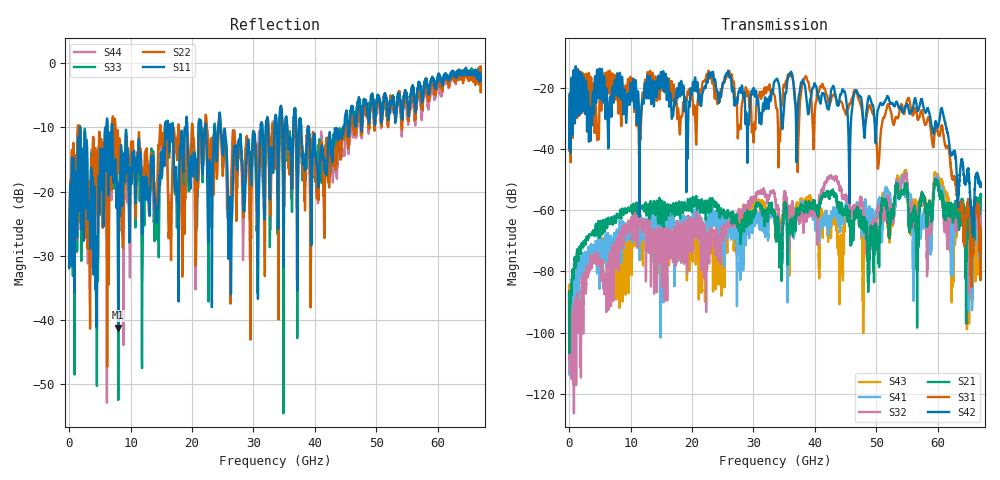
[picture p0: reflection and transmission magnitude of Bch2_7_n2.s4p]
!Agilent Technologies,N5247A,US51170199,A.09.90.13
!Agilent N5247A: A.09.90.13
!Date: Wednesday, October 17, 2018 18:12:49
!Correction: S11(Full 4 Port(1,2,3,4))
!S12(Full 4 Port(1,2,3,4))
!S13(Full 4 Port(1,2,3,4))
!S14(Full 4 Port(1,2,3,4))
!S21(Full 4 Port(1,2,3,4))
!S22(Full 4 Port(1,2,3,4))
!S23(Full 4 Port(1,2,3,4))
!S24(Full 4 Port(1,2,3,4))
!S31(Full 4 Port(1,2,3,4))
!S32(Full 4 Port(1,2,3,4))
!S33(Full 4 Port(1,2,3,4))
!S34(Full 4 Port(1,2,3,4))
!S41(Full 4 Port(1,2,3,4))
!S42(Full 4 Port(1,2,3,4))
!S43(Full 4 Port(1,2,3,4))
!S44(Full 4 Port(1,2,3,4))
!S4P File: Measurements: <S11,S12,S13,S14>,
!<S21,S22,S23,S24>,
!<S31,S32,S33,S34>,
!<S41,S42,S43,S44>:
# Hz S  dB  R 50
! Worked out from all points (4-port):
!   6701 points, 10 MHz to 67 GHz, reference 50 ohm
!   strongest paths, dB at 10 MHz, 16.76 GHz, 33.51 GHz, 50.25 GHz, 67 GHz:
!     S42: -39.6, -29.6, -17.7, -27.3, -52.3
!     S31: -40.5, -21.3, -23.2, -46.1, -70.7
!     S21: -86.6, -61.3, -63.4, -72.0, -55.8
!     S32: -87.6, -68.3, -56.3, -60.9, -61.9
!     S41: -87.3, -70.5, -63.2, -57.5, -73.4
!     S43: -84.4, -75.3, -64.1, -61.4, -66.6
!   lowest |S11| = -41.2 dB at 7.999 GHz (marker M1), VSWR 1.02, Z = 49.4 + j0.663 ohm
!   |S11| at or under -10 dB: 7.041 GHz to 15.66 GHz (8.62 GHz wide, 75.9 % of centre); 24.66 GHz to 31.15 GHz (6.492 GHz wide, 23.3 % of centre); 38.96 GHz to 44.63 GHz (5.664 GHz wide, 13.6 % of centre)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
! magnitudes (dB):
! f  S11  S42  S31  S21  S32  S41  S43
! 10 MHz  -31.7  -39.6  -40.5  -86.6  -87.6  -87.3  -84.4
! 7.999 GHz  -41.2  -19.2  -28.0  -62.7  -73.8  -73.3  -69.5
! 34.16 GHz  -11.2  -19.1  -36.1  -72.1  -62.3  -66.9  -62.7
! 38.44 GHz  -16.2  -20.3  -16.5  -58.1  -60.7  -59.2  -56.9
! 50.32 GHz  -5.1  -26.9  -45.4  -74.0  -59.6  -57.5  -62.1
! 55.19 GHz  -6.9  -26.5  -23.4  -60.1  -55.4  -55.0  -59.7
! 67 GHz  -2.7  -52.3  -70.7  -55.8  -61.9  -73.4  -66.6
